(* Logix 5000 AddOnInstructionDefinition export Banner_RSio_Fault_Info_v1; software revision 33.00 *)

TYPE Banner_RSio_ISD_Fault_v1 :
STRUCT
   Operation : SINT;   // 1=Input Fault, 2=Output Fault, 3=TP Fault
   Point : SINT;   // Value of the point to access the fault for. Inputs have 0 to 11 points, Outputs have 0 to 3, and TP have 0 to 11.
   FaultInfo : SINT[8];
END_STRUCT
END_TYPE

ADD_ON_INSTRUCTION Banner_RSio_Fault_Info_v1   (* revision 1.0 *)
VAR_IN_OUT
   Fault : Banner_RSio_ISD_Fault_v1; {required}
   MSG : MESSAGE; {required}
   Activate : BOOL; {required}
END_VAR
VAR_OUTPUT
   Busy : BOOL; {visible}
   Done : BOOL; {visible}
   Error : BOOL; {visible}
END_VAR
VAR
   Timer : TIMER := (PRE := 5000); {access None}
   Control : DINT; {access None}
END_VAR

ROUTINE Logic   (* ladder *)
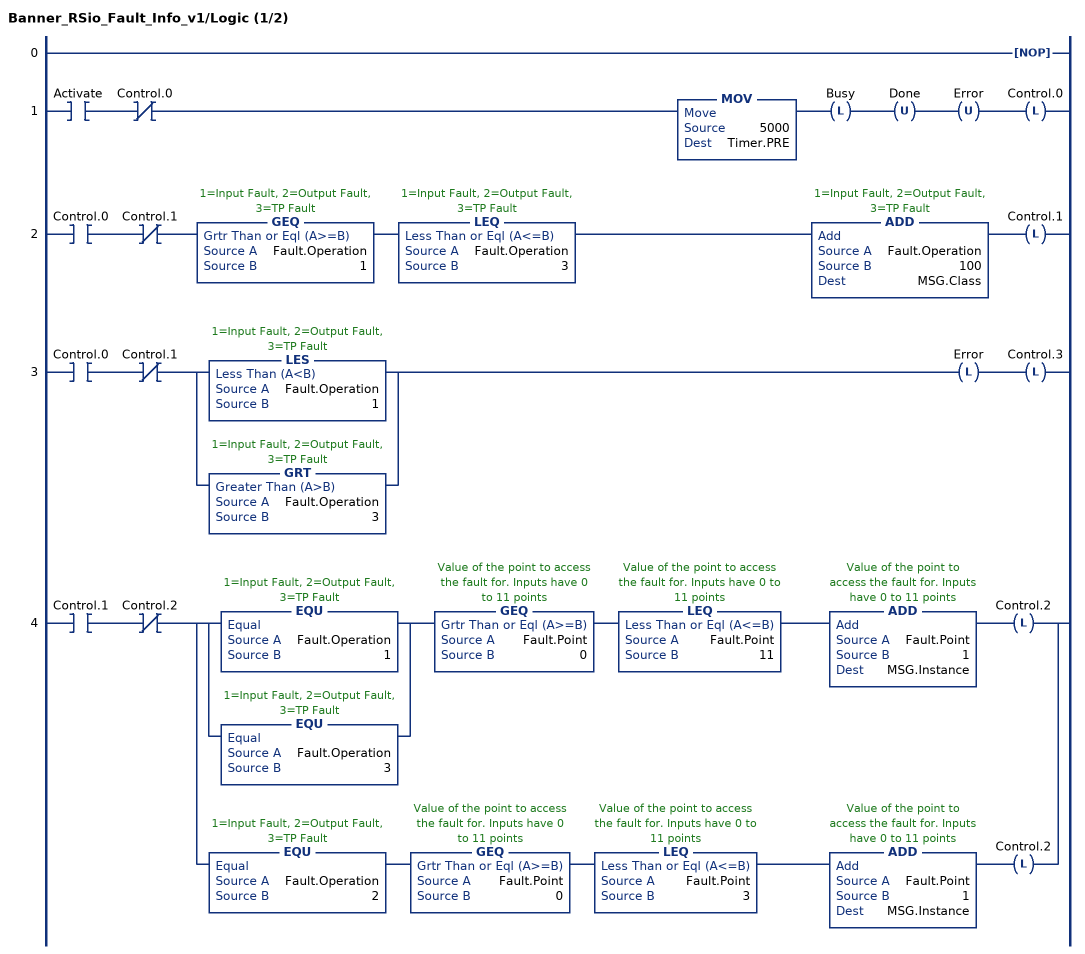
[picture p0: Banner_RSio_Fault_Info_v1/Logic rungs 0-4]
   0: NOP();
   1: XIC(Activate)XIO(Control.0)MOV(5000,Timer.PRE)OTL(Busy)OTU(Done)OTU(Error)OTL(Control.0);
   2: XIC(Control.0)XIO(Control.1)GEQ(Fault.Operation,1)LEQ(Fault.Operation,3)ADD(Fault.Operation,100,MSG.Class)OTL(Control.1);
   3: XIC(Control.0)XIO(Control.1)[LES(Fault.Operation,1) ,GRT(Fault.Operation,3) ]OTL(Error)OTL(Control.3);
   4: XIC(Control.1)XIO(Control.2)[[EQU(Fault.Operation,1) ,EQU(Fault.Operation,3) ] GEQ(Fault.Point,0) LEQ(Fault.Point,11) ADD(Fault.Point,1,MSG.Instance) OTL(Control.2) ,EQU(Fault.Operation,2) GEQ(Fault.Point,0) LEQ(Fault.Point,3) ADD(Fault.Point,1,MSG.Instance) OTL(Control.2) ];
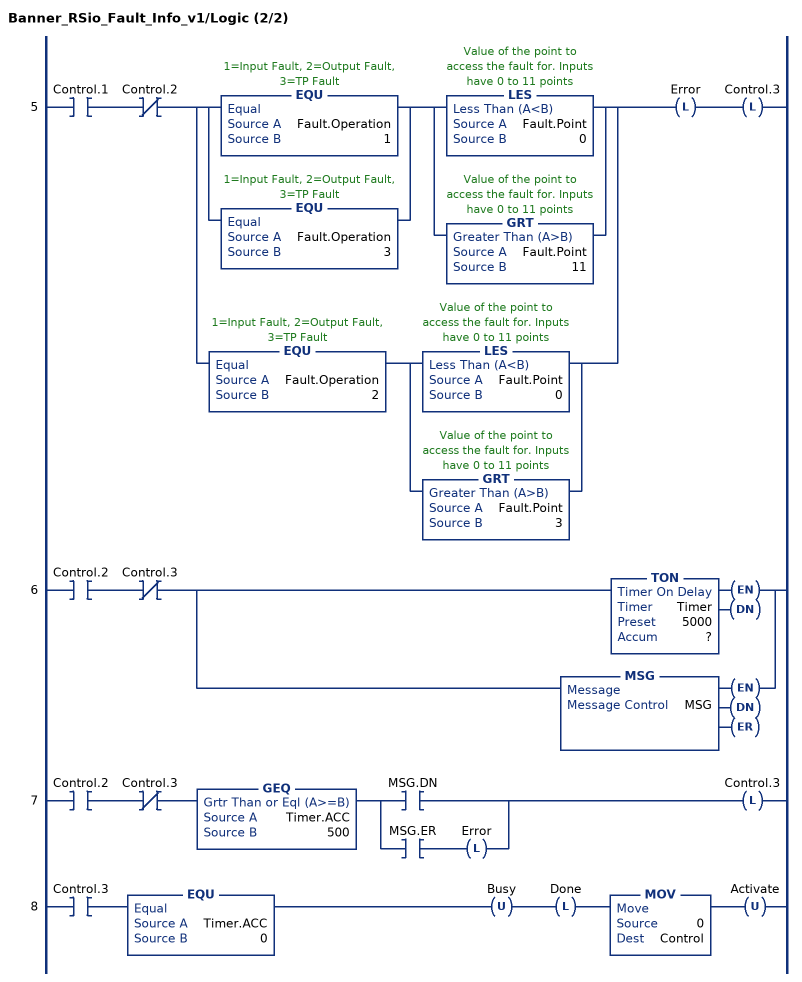
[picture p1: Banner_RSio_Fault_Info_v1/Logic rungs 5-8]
   5: XIC(Control.1)XIO(Control.2)[[EQU(Fault.Operation,1) ,EQU(Fault.Operation,3) ] [LES(Fault.Point,0) ,GRT(Fault.Point,11) ] ,EQU(Fault.Operation,2) [LES(Fault.Point,0) ,GRT(Fault.Point,3) ] ]OTL(Error)OTL(Control.3);
   6: XIC(Control.2)XIO(Control.3)[TON(Timer,?,?) ,MSG(MSG) ];
   7: XIC(Control.2)XIO(Control.3)GEQ(Timer.ACC,500)[XIC(MSG.DN) ,XIC(MSG.ER) OTL(Error) ]OTL(Control.3);
   8: XIC(Control.3)EQU(Timer.ACC,0)OTU(Busy)OTL(Done)MOV(0,Control)OTU(Activate);
END_ROUTINE
END_ADD_ON_INSTRUCTION
